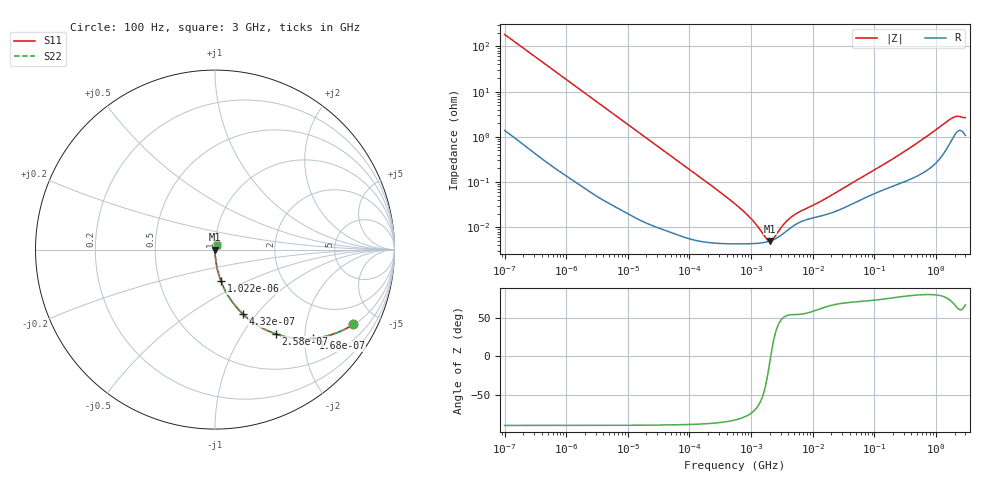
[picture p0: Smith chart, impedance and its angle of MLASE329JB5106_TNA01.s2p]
! MLASE329JB5106_TNA01  S-PARAMETER MODEL  ( Standard Model )
! Model Generated by TAIYO YUDEN Corporation (http://www.ty-top.com)
! Version 1.0
! TAIYO YUDEN Control No. 220601
! Copyright(c) 2009 TAIYO YUDEN CO.,LTD. All Rights Reserved.
! Product Description (link to TY-COMPAS)
! https://ds.yuden.co.jp/TYCOMPAS/or/detail?pn=MLASE329JB5106KTNA01&u=M
! Products Name : Multilayer Ceramic Capacitors
! Characteristics :
!  Capacitance : 10 [uF] , Rated Voltage : 16 [V] , TCC : X5R
!  Case Size : 3.2 x 2.5 / 0.126 x 0.098 [mm/inch] , Thickness : 0.85 / 0.033 [mm/inch]
!  (Conditions: Temperature = 25 [degC] , DC Bias Voltage = 0 [V])
! External Node Assignments :
!  1  o---| |---o  2
! GND o---------o GND
! Frequency Range : 100Hz  -  3GHz  [ 401 STEP ]
# MHZ S RI R 50
! Freq[MHz].  S11 Real  S11 Imag  S21 Real  S21 Imag  S12 Real  S12 Imag  S22 Real  S22 Imag
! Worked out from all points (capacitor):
!   401 points, 100 Hz to 3 GHz, reference 50 ohm
!   read as one part in series: C = 8.65 uF near 109 Hz
!   lowest |Z| = 4.99 mohm at 1.992 MHz (marker M1)
!   series resonance near 2.084 MHz, so ESL is about 670 pH
!   S11 on the Smith chart (normalised r, x): 100 Hz: 1.03, -3.68; 168 Hz: 1.02, -2.20; 258 Hz: 1.01, -1.43; 432 Hz: 1.01, -0.86; 1.022 kHz: 1.00, -0.36; 3 GHz: 1.02, +0.05
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0.0001  0.7699 -0.4172  0.2301 0.4172  0.2301 0.4172  0.7699 -0.4172
0.000168  0.547 -0.4941  0.453 0.4941  0.453 0.4941  0.547 -0.4941
0.000258  0.3403 -0.4702  0.6597 0.4702  0.6597 0.4702  0.3403 -0.4702
0.000432  0.1568 -0.3601  0.8432 0.3601  0.8432 0.3601  0.1568 -0.3601
0.000636  0.0798 -0.2675  0.9202 0.2675  0.9202 0.2675  0.0798 -0.2675
0.001022  0.0332 -0.1755  0.9668 0.1755  0.9668 0.1755  0.0332 -0.1755
0.001788  0.0115 -0.1029  0.9885 0.1029  0.9885 0.1029  0.0115 -0.1029
0.005476  0.00148 -0.0341  0.9985 0.0341  0.9985 0.0341  0.00148 -0.0341
0.031977  0.000131 -0.00591  0.9999 0.00591  0.9999 0.00591  0.000131 -0.00591
0.547723  4.29e-05 -0.000326  1 0.000326  1 0.000326  4.29e-05 -0.000326
0.842342  4.29e-05 -0.000191  1 0.000191  1 0.000191  4.29e-05 -0.000191
1.295438  4.42e-05 -9.17e-05  1 9.17e-05  1 9.17e-05  4.42e-05 -9.17e-05
1.411895  4.47e-05 -7.43e-05  1 7.43e-05  1 7.43e-05  4.47e-05 -7.43e-05
1.992254  4.92e-05 -8.39e-06  1 8.39e-06  1 8.39e-06  4.92e-05 -8.39e-06
3.063887  6.66e-05 7.16e-05  0.9999 -7.16e-05  0.9999 -7.16e-05  6.66e-05 7.16e-05
4.91919  0.000108 0.000149  0.9999 -0.000149  0.9999 -0.000149  0.000108 0.000149
9.794414  0.000159 0.000254  0.9998 -0.000254  0.9998 -0.000254  0.000159 0.000254
175.1444  0.00076 0.00282  0.9992 -0.00282  0.9992 -0.00282  0.00076 0.00282
513.708  0.00145 0.00741  0.9986 -0.00741  0.9986 -0.00741  0.00145 0.00741
1789.813  0.0089 0.0238  0.9911 -0.0238  0.9911 -0.0238  0.0089 0.0238
2219.584  0.0135 0.0247  0.9865 -0.0247  0.9865 -0.0247  0.0135 0.0247
3000  0.0112 0.0239  0.9888 -0.0239  0.9888 -0.0239  0.0112 0.0239
